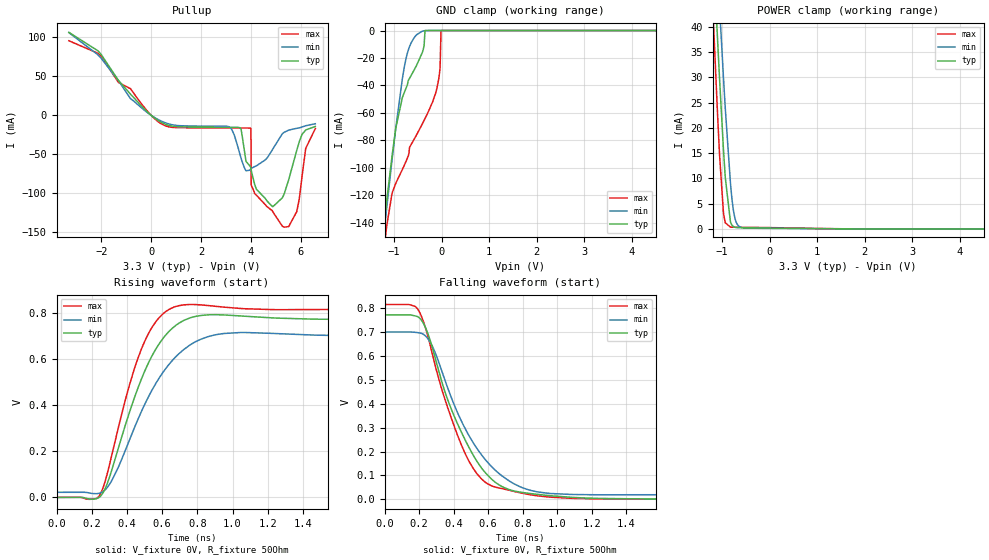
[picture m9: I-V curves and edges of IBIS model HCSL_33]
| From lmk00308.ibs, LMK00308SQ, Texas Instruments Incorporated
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|   Model HCSL_33
[Model]   HCSL_33
Model_type   Open_source
Polarity   Non-Inverting
Rref =   50.0000
Vref =   1.65
Vmeas =   1.65
|   typ   min   max
C_comp   1.5032pF   1.4574pF   1.5495pF
|Output in low   Nom   Weak   Strong
|C_Comp   1.5032pF   1.4574pF   1.5495pF
|Output in High   Nom   Strong   Weak
|C_Comp   1.0889pF   1.0724pF   1.10585pF
[Voltage Range]   3.3   3.125   3.465
[Temperature Range]   45   125   -40
[Pullup Reference]   3.3   3.125   3.465
[Pulldown Reference]   0   0   0
[Power Clamp Reference]   3.3   3.125   3.465
[GND Clamp Reference]   -0   0   -0
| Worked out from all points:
|   slope of the pullup table from 0 to 0.495 V, typ, clamps not added: 47.8 ohm
|   GND clamp passes 1 mA (typ) near -0.35 V on its own axis
|   POWER clamp passes 1 mA (typ) near -0.81 V on its own axis
|   falling waveform, V_fixture 0V, R_fixture 50Ohm: 20-80 % time 256ps typ, 276ps min, 225ps max; typ from 0.773 V to 0 V
|   rising waveform, V_fixture 0V, R_fixture 50Ohm: 20-80 % time 217ps typ, 260ps min, 180ps max; typ from 0 V to 0.773 V
[GND Clamp]
|   Voltage   I(typ)   I(min)   I(max)
-3.3V     -1.043A    -996.1mA   -1.089A
-1.211V   -141.1mA   -147.5mA   -159.3mA
-1.162V   -126mA     -131.4mA   -144.5mA
-963.6mV  -70.9mA    -70.87mA   -111.2mA
-785.4mV  -45.14mA   -26.66mA   -98.18mA
-636.9mV  -32.43mA   -8.721mA   -82.8mA
-409.2mV  -16.23mA   -510.4uA   -68.24mA
-349.8mV  0A         -134.1uA   -64.14mA
-102.3mV  0A         -237.5nA   -42.45mA
-33mV     0A         -16.69nA   -26.95mA
-13.2mV   0A         -210.4pA   0A
6.59V     0A         0A         0A
[Pullup]
|   Voltage   I(typ)   I(min)   I(max)
-3.3V     106.2mA    105.9mA    95.43mA
561mV     -11.36mA   -9.555mA   -13.37mA
3.135V    -15.48mA   -14.92mA   -16.33mA
3.571V    -16.04mA   -50.73mA   -16.34mA
3.996V    -66.51mA   -69.03mA   -16.77mA
4.006V    -68.24mA   -68.72mA   -17.15mA
4.016V    -69.95mA   -68.43mA   -89.43mA
4.867V    -116.8mA   -44.31mA   -122.4mA
5.343V    -100.6mA   -21.79mA   -143.4mA
5.848V    -44.67mA   -16.72mA   -122.9mA
6.204V    -18.84mA   -13.42mA   -42.48mA
6.59V     -14.36mA   -10.91mA   -17mA
[POWER Clamp]
|   Voltage   I(typ)   I(min)   I(max)
-3.3V     591mA      563.1mA    632.3mA
-1.191V   56mA       69.05mA    42.73mA
-1.102V   38.65mA    52.49mA    23.91mA
-1.053V   29.47mA    43.66mA    14.46mA
-973.5mV  15.96mA    30.2mA     3.365mA
-933.9mV  10.18mA    23.88mA    1.219mA
-825mV    1.397mA    9.072mA    360.5uA
-775.5mV  581.4uA    4.543mA    346.4uA
-726mV    327.7uA    1.963mA    341.4uA
-666.6mV  254.2uA    731.6uA    336.4uA
-557.7mV  234.9uA    210uA      326.9uA
6.59V     0A         0A         0A
[Ramp]
R_load = 50
|   typ   min   max
dV/dt_r   0.463882/2.16874e-10   0.407428/2.59996e-10   0.490159/1.79628e-10
dV/dt_f   0.463574/2.55644e-10   0.407643/2.75523e-10   0.489651/2.24741e-10
[Falling Waveform]
V_fixture = 0V
V_fixture_min = 0V
V_fixture_max = 0V
R_fixture = 50Ohm
C_fixture = 0F
|   Time   V(typ)   V(min)   V(max)
0s        772.7mV    700.9mV    816.1mV
195ps     763.5mV    697.8mV    793.3mV
275ps     639.6mV    643.7mV    613.7mV
360ps     428.7mV    477.8mV    396mV
450ps     273.7mV    320.2mV    219.3mV
535ps     159.1mV    212.9mV    107.4mV
625ps     81.09mV    133.3mV    55.12mV
785ps     30.11mV    52.5mV     27.3mV
965ps     14.86mV    24.23mV    8.814mV
2.99ns    35.8uV     21.5mV     7.815uV
[Rising Waveform]
V_fixture = 0V
V_fixture_min = 0V
V_fixture_max = 0V
R_fixture = 50Ohm
C_fixture = 0F
|   Time   V(typ)   V(min)   V(max)
0s        5.846uV    22.11mV    14.88nV
245ps     1.907mV    18.69mV    9.539mV
315ps     121.6mV    74.76mV    187.3mV
410ps     359.7mV    241mV      476.7mV
480ps     509.8mV    369.5mV    640.1mV
570ps     651.7mV    502.5mV    768.6mV
670ps     742.6mV    604.9mV    827.2mV
820ps     790.1mV    687mV      836mV
1.045ns   788.1mV    716.1mV    820.5mV
2.99ns    773.1mV    701.2mV    816.9mV
